(* 	
	Program Name: 	ACS_CMD_SOFTWARE_STOP
	Purpose:		Copy Software Stop (ESTOP) Command to ACS Drive Output Command Register
	When Executed:	Performs action defined for Software Stop (in TMI)
*)
PROGRAM ACS_CMD_SOFTWARE_STOP
VAR_IN_OUT
	Axis:ACS_DRIVE_TYPE;
END_VAR
VAR
	_command:	USINT	:= ACS_COMMANDS.SOFTWARE_STOP;
END_VAR

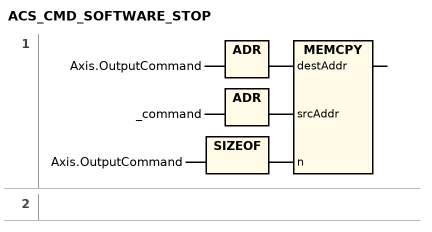
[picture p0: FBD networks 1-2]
// NETWORK 1
MEMCPY(destAddr := ADR(Axis.OutputCommand), srcAddr := ADR(_command), n := SIZEOF(Axis.OutputCommand));

// NETWORK 2

END_PROGRAM
